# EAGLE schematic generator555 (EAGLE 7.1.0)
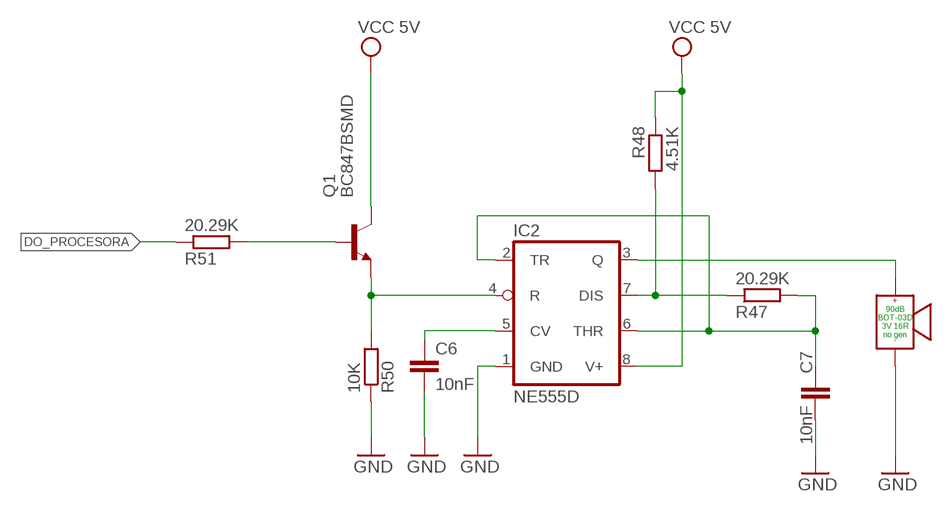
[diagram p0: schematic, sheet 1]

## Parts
C6  10nF  C-EUC0805  [C0805]
C7  10nF  C-EUC0805  [C0805]
IC2  NE555D  [SO08]
Q1  BC847BSMD  [SOT23]
R47  20.29K  R-EU_R0805  [R0805]
R48  4.51K  R-EU_R0805  [R0805]
R50  10K  R-EU_R0805  [R0805]
R51  20.29K  R-EU_R1206  [R1206]
U$20  BOT-03D  [BOT-03D]

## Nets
DO-BUZZER: R51.1
GND: C6.2 C7.2 IC2.1(GND) R50.1 U$20.PM
N$40: IC2.4(R) Q1.2(E) R50.2
N$44: Q1.1(B) R51.2
N$85: C6.1 IC2.5(CV)
N$86: IC2.3(Q) U$20.PP
N$87: C7.1 IC2.2(TR) IC2.6(THR) R47.2
N$88: IC2.7(DIS) R47.1 R48.2
VCC: IC2.8(V+) Q1.3(C) R48.1 ; supply symbol labelled VCC 5V

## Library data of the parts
C6 C7 = rcl:C-EU: CAPACITOR, European symbol
IC2 = _adafruit:*555: TIMER Changed DIP package to have round (not oval) pin pads http://www.ladyada.net/library/pcb/eaglelibrary.html
Q1 = transistor-npn:BC847*: NPN Transistor
R47 R48 R50 R51 = rcl:R-EU_: RESISTOR, European symbol
U$20 = .Moje:BOT-03D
